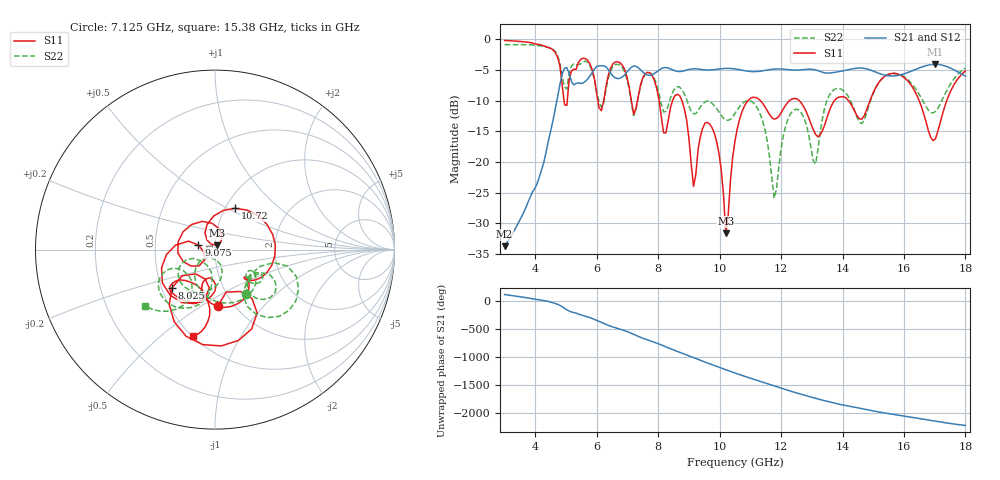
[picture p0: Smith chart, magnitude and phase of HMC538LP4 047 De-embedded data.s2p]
! Chelmsford, MA 01824
! http://www.hittite.com
! Tel: 978-250-3343
! Fax: 978-250-3373
! Device  :  HMC538LP4
! Description:  600 Analog Phase Shifter
! Frequency  :  6.0 GHz - 15.0 GHz
! Package  :  LP4  - 4x4 mm Quad Flatpack No-Lead (QFN) Plastic Package: 24 pin
! Ports  :  2 RF, 1 DC
!  Pin  3  = Rfin  = Port 1
!  Pin  16  = Rfout = Port 2
!  pin  21  = vCTL
! Voltages:  VCTL  = 0 to 5.0 Volts
! Currents :  Vb(V)  Vd(V)  Ib(mA)  Id(mA)
!  0.00  4.70  0.000000	0.491120
! Data:  The device was measured on evaluation board 111296-1.
!  Data was collected using a calibrated network analyzer.
!  The evaluation circuit board was modeled and simulated.This was use
!  to removed the evaluation board circuit from the measured data.
!  The reference plane is the center of the package pin.
! Misc:  Lot #
!Date Measured:  03 - 11 -2009
! Date:  03 - 17 -2009
! Note:
!  Hittite Microwave supplies this data as a sample of measured data at the
!  package pin for this package product.  Your particular data for this product
!  may vary.
!  Data was taken at 25 degrees C.
!  Hittite Microwave reserves the right to change this data at anytime.
# MHz S MA R 50
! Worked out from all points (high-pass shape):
!   201 points, 3 GHz to 18 GHz, reference 50 ohm
!   highest |S21| = -4.08 dB at 17.02 GHz (marker M1); lowest = -33.7 dB at 3 GHz (marker M2)
!   |S21| within 3 dB of the highest: 4.813 GHz to 5.203 GHz (389.6 MHz wide, 7.78 % of centre); 5.566 GHz to end of sweep
!   lowest |S11| = -31.6 dB at 10.2 GHz (marker M3), VSWR 1.05, Z = 50.9 + j2.49 ohm
!   |S11| at or under -10 dB: 8.772 GHz to 10.92 GHz (2.152 GHz wide, 21.9 % of centre); 11.33 GHz to 12.28 GHz (947 MHz wide, 8.02 % of centre); 12.59 GHz to 13.74 GHz (1.144 GHz wide, 8.69 % of centre)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
!   |S22| runs from -25.9 to -0.9 dB; largest |S21 - S12| = 0.0025
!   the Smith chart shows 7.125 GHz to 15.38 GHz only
!   S11 on the Smith chart (normalised r, x): 7.125 GHz: 0.84, -0.59; 8.025 GHz: 0.57, -0.27; 9.075 GHz: 0.83, +0.04; 10.72 GHz: 1.11, +0.55; 15.38 GHz: 0.50, -0.65
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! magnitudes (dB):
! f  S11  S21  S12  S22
! 3 GHz  -0.2  -33.7  -33.7  -0.9
! 4.575 GHz  -1.7  -13.2  -13.2  -1.6
! 4.95 GHz  -10.7  -4.7  -4.7  -7.7
! 5.55 GHz  -3.1  -7.1  -7.1  -3.8
! 7.125 GHz  -10.0  -4.6  -4.6  -10.3
! 8.025 GHz  -9.9  -5.0  -5.0  -8.8
! 8.7 GHz  -9.2  -5.3  -5.3  -7.8
! 9.075 GHz  -20.4  -4.9  -4.9  -11.8
! 9.75 GHz  -14.4  -5.0  -5.0  -10.4
! 10.2 GHz  -31.6  -4.7  -4.8  -13.2
! 10.5 GHz  -16.6  -4.8  -4.8  -12.1
! 10.72 GHz  -11.8  -5.0  -5.0  -10.5
! 11.4 GHz  -10.4  -5.1  -5.2  -13.3
! 11.78 GHz  -13.0  -4.9  -4.9  -25.9
! 12.38 GHz  -9.7  -5.0  -5.0  -11.7
! 13.05 GHz  -14.8  -4.9  -4.9  -19.8
! 13.65 GHz  -10.7  -5.5  -5.5  -8.5
! 14.62 GHz  -13.0  -4.7  -4.7  -13.7
! 15.38 GHz  -6.0  -5.8  -5.9  -6.0
! 15.53 GHz  -5.7  -6.0  -6.0  -5.7
! 17.02 GHz  -16.2  -4.1  -4.1  -11.8
! 18 GHz  -5.2  -6.0  -6.0  -4.7
